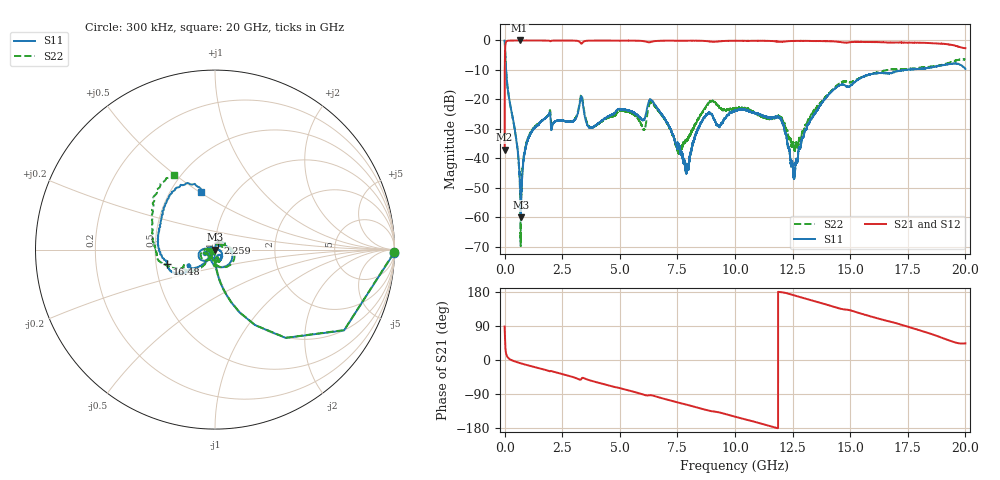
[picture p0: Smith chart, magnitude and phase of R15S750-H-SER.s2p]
!{R15S750}
!Johanson Technology Inc.
!www.johansontechnology.com
!Test Board Conditions:
!Substrate Type  RO4350B
!Substrate Thickness  20 mil
!Substrate Dk  3.66
!TL Type: GCPW
!TL Trace Width  34 mil
!TL Gap  10 mil
!Electrode orientation  Horizontal
!DUT TOPOLOGY	SERIES
!Mounting Pad LxW  26x52 mil
! Created Sat Feb  6 14:36:08 2021
# hz S ma R 50
! 2 Port Network Data from SP1.SP block
! freq  magS11  angS11  magS21  angS21  magS12  angS12  magS22  angS22
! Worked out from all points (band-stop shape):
!   20001 points, 300 kHz to 20 GHz, reference 50 ohm
!   highest |S21| = 0.00 dB at 648.3 MHz (marker M1); lowest = -37.1 dB at 300 kHz (marker M2)
!   |S21| within 3 dB of the highest: 21.46 MHz to end of sweep
!   lowest |S11| = -60.0 dB at 701.3 MHz (marker M3), VSWR 1.00, Z = 49.9 + j0.012 ohm
!   |S11| at or under -10 dB: 63.51 MHz to 17.36 GHz (17.3 GHz wide, 199 % of centre); 17.35942 GHz to 17.37336 GHz (13.94 MHz wide, 0.0803 % of centre); 17.37499 GHz to 17.41082 GHz (35.84 MHz wide, 0.206 % of centre)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
!   |S22| runs from -69.9 to 0.0 dB; largest |S21 - S12| = 0.017
!   S11 on the Smith chart (normalised r, x): 300 kHz: open; 2.259 GHz: 1.03, +0.08; 16.48 GHz: 0.57, -0.10; 20 GHz: 0.71, +0.51
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300000  0.9978 -1.0  0.01402 88.5  0.01409 89.1  0.9975 -0.9
1.123e8  0.1835 -81.0  0.9826 9.0  0.9825 9.0  0.1836 -80.7
6.483e8  0.005294 -108.3  0.9999 -7.8  0.9989 -7.8  0.004908 -92.3
7.013e8  0.001 173.1  0.9999 -8.8  0.999 -8.8  0.000543 38.4
1.1413e9  0.02671 78.8  0.9983 -16.1  0.999 -16.1  0.02802 71.5
2.2593e9  0.04335 64.9  0.9972 -33.3  0.9973 -33.3  0.04288 46.2
2.9853e9  0.04239 44.7  0.994 -45.4  0.9944 -45.3  0.0434 32.6
3.3343e9  0.1124 -48.6  0.8826 -49.7  0.883 -49.6  0.1216 -39.7
3.7603e9  0.03279 -141.5  0.9939 -54.8  0.9944 -54.7  0.03375 -130.5
6.0363e9  0.04465 -144.6  0.9739 -91.5  0.9748 -91.5  0.03072 -151.7
6.6673e9  0.06763 178.2  0.984 -98.0  0.9844 -98.0  0.06386 -176.7
7.5423e9  0.01695 163.2  0.9897 -112.5  0.9896 -112.5  0.01288 -154.2
7.9093e9  0.006878 84.9  0.989 -118.1  0.9885 -118.0  0.02017 -100.6
8.7083e9  0.05096 -37.3  0.9795 -131.3  0.9789 -131.3  0.07059 -72.3
1.00003e10  0.0643 -59.3  0.9865 -149.5  0.9866 -149.5  0.06945 -74.0
1.19293e10  0.04801 -161.7  0.9491 179.4  0.9514 179.5  0.05202 -126.9
1.25263e10  0.006562 -169.0  0.9801 171.4  0.9802 171.4  0.01863 -168.1
1.33343e10  0.04762 -123.3  0.9795 157.3  0.9793 157.3  0.05742 -120.2
1.44673e10  0.1673 -141.6  0.9529 137.2  0.9521 137.1  0.1763 -137.1
1.64803e10  0.2782 -163.1  0.9282 105.0  0.9213 105.1  0.3068 -166.3
1.66673e10  0.2738 -166.4  0.9225 102.1  0.9086 102.0  0.3201 -168.6
2e10  0.3279 103.3  0.7388 43.8  0.7302 43.8  0.4722 118.8
